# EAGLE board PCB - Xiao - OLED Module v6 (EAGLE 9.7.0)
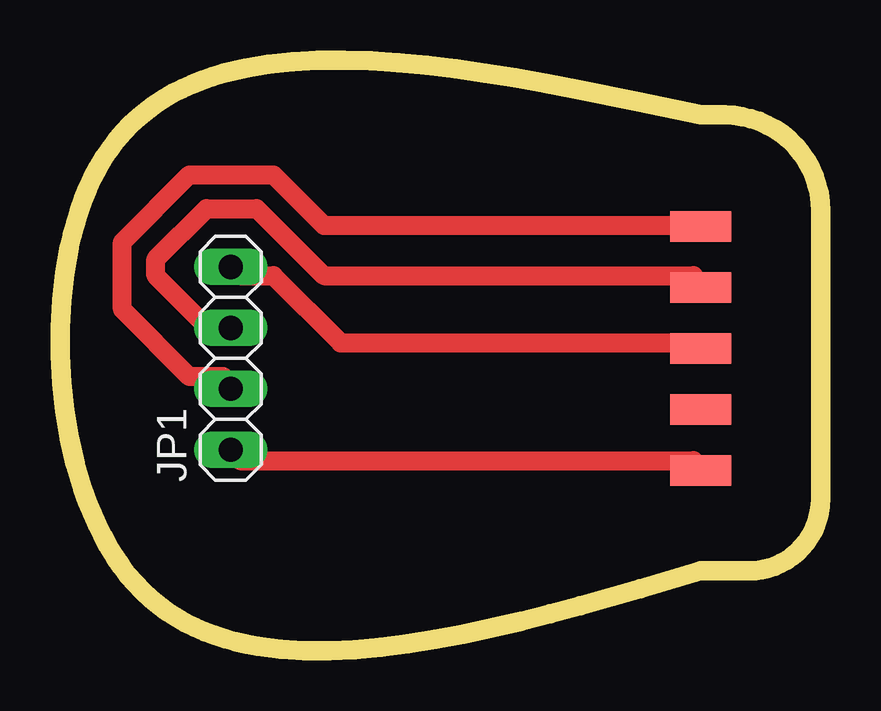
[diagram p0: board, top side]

Size 31.69 x 24.62 mm. Coordinates in mm from the lower left corner, seen from the top.
Outline: 87 segments
Copper layers (1*16): Top 0.035mm / dielectric 1.5mm / Bottom 0.035mm
Design rules "fab.dru": minimum track width 0.8mm, minimum drill 32mil, track to track 0.6mm, track to pad 0.6mm, pad to pad 0.6mm, via to via 0.6mm, smd to smd 6mil, copper to edge 16mil, drill to drill 16mil, minimum pad ring 10mil, minimum via ring 8mil, stop-mask expansion 4mil, vias tented up to drill 0mil, thermal gap 16mil

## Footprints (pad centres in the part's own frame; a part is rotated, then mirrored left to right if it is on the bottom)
1X04 = drill 1.016 long: 1 -3.81,0; 2 -1.27,0; 3 1.27,0; 4 3.81,0
1X05SMD = smd 2.54 x 1.27: 1 0,6.35; 2 0,3.81; 3 0,1.27; 4 0,-1.27; 5 0,-3.81

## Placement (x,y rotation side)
JP1  PINHD-1X4  [1X04]  7.11,12.19 90 top
U$1  1X5_PAD_SMD  [1X05SMD]  26.69,11.33 0 top

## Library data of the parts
JP1 = Connector; CATEGORY: Headers; DESCRIPTION: Header-Straight-4 Position; PACKAGE_TYPE: THT; PITCH: 0.100" (2.54mm); SUBCATEGORY: Headers-Male Pins; TYPE: Board to Board or Cable-Unshrouded-Through Hole-Straight
U$1 = Carl_Lib

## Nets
N$1: JP1.1 U$1.5
N$2: JP1.2 U$1.1
N$3: JP1.3 U$1.2
N$4: JP1.4 U$1.3

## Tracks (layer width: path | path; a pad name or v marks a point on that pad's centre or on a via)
N$1
  Top 0.8: U$1.5 26.39,7.93 7.49,7.93 JP1.1
N$2
  Top 0.8: U$1.1 26.39,17.73 10.99,17.73 8.89,19.83 5.39,19.83 2.59,17.03 2.59,14.23 5.39,11.43 6.79,11.43 JP1.2
N$3
  Top 0.8: U$1.2 26.39,15.63 10.99,15.63 8.19,18.43 6.09,18.43 3.99,16.33 3.99,15.63 6.09,13.53 6.79,13.53 JP1.3
N$4
  Top 0.8: U$1.3 26.39,12.83 11.69,12.83 8.89,15.63 7.49,15.63 JP1.4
